PROGRAM MAIN_CM
VAR CONSTANT
	(* init-pars *)
	cInitPars	: ST_CM_SpikeEnergySpectrum_InitPars :=(	nFFT_Length				:= cFFTLength,
															nWindowLength			:= cWindowLength,
															fSamplerate				:= cSampleRate,
															fDecayTime				:= cDecayTime,
															fLowerFrequencyLimit	:= cLowerFrequencyLimit,
															fUpperFrequencyLimit	:= cUpperFrequencyLimit,
															nOrder					:= cOrder,
															aWindowParameters		:= cWindowParameters,
															eWindowType				:= cWindowType,
															nOverlap				:= cOverlap,
															eScalingType			:= cScalingType,
															bTransformToDecibel		:= cTransformToDecibel);
END_VAR
VAR
	fbSESpectrum	: FB_CMA_SpikeEnergySpectrum := ( stInitPars := cInitPars, nOwnID := eID_SESpectrum, aDestIDs := [eID_Sink] );
	
	bConfigure 		: BOOL := TRUE;
	aConfigParams	: ARRAY [1..3] OF LREAL;
END_VAR

(* Call Spike Energy Spectrum Configure *)
IF bConfigure THEN
	// Set parameters
	aConfigParams[1] := cDecayTime;					// T_def, i.e. time between peaks in samples [1]; e.g. cDefectFrequency / cResolution.
	aConfigParams[2] := cLowerFrequencyLimit;		// Highpass frequency of bandpass filter [Hz]
	aConfigParams[3] := cUpperFrequencyLimit;		// Lowpass frequency of bandpass filter [Hz] 
	
	// Call
	fbSESpectrum.Configure(pArg:=ADR(aConfigParams), nArgSize:=SIZEOF(aConfigParams));
	IF fbSESpectrum.bError THEN
		fbErrHist.AddError(bErr:=TRUE, hrErrCode:=fbSESpectrum.hrErrorCode, sErrSource:='MAIN_CM.fbSESpectrum.Configure'); // error monitoring
		// ToDo: if error
	ELSE
		bConfigure := FALSE;
	END_IF
END_IF

(* Call Spike Energy Spectrum Call *)
fbSESpectrum.Call();
IF fbSESpectrum.bError THEN
	fbErrHist.AddError(bErr:=TRUE, hrErrCode:=fbSESpectrum.hrErrorCode, sErrSource:='MAIN_CM.fbSESpectrum.Call'); // error monitoring
	// ToDo: if error
END_IF

END_PROGRAM
